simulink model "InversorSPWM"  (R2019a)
settings: Solver=ode23t  StartTime=0.0  StopTime=0.06  RelTol=1e-3
libraries: powerlib x22, powerlib_meascontrol x5, simulink x4

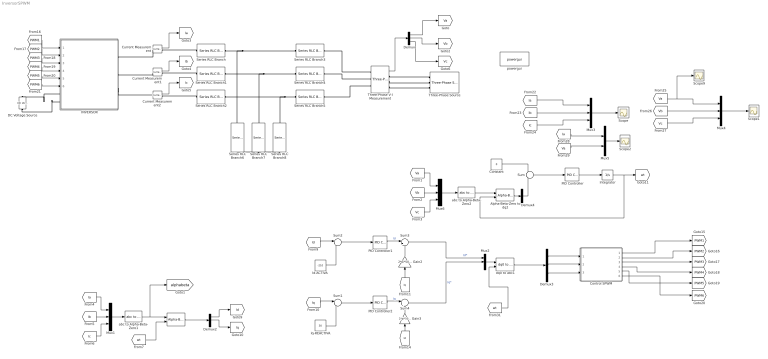
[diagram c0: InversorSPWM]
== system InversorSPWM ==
  " " : powerlib_meascontrol/Transformations/Alpha-Beta-Zero to dq0  Alignment=90 degrees behind phase A axis
  Alpha-Beta-Zero to dq2 : powerlib_meascontrol/Transformations/Alpha-Beta-Zero to dq0  Alignment=90 degrees behind phase A axis
  Constant : Constant  Value=0
  "Control SPWM " : Subsystem
  Current Measurement : powerlib/Measurements/Current Measurement  PhasorSimulation=off  OutputType=Complex  PSBequivalent=0
  Current Measurement1 : powerlib/Measurements/Current Measurement  PhasorSimulation=off  OutputType=Complex  PSBequivalent=0
  Current Measurement2 : powerlib/Measurements/Current Measurement  PhasorSimulation=off  OutputType=Complex  PSBequivalent=0
  DC Voltage Source : powerlib/Electrical Sources/DC Voltage Source  Amplitude=800  Measurements=None
  Demux{,2..4} (4 alike) : Demux  Outputs=3
  Gain2 : Gain  Gain=2*pi*50*1000e-6
  Gain3 : Gain  Gain=2*pi*50*1000e-6
  INVERSOR : Subsystem
  "Id-ACTIVA " : Constant  Value=-210
  Integrator : Integrator
  Iq-REACTIVA : Constant  Value=30
  Mux{1..4,6} (5 alike) : Mux  Inputs=3
  Mux5 : Mux  Inputs=2
  PID Controller : simulink/Continuous/PID Controller  Controller=PI  Form=Parallel  TimeDomain=Continuous-time  SampleTime=-1  IntegratorMethod=Forward Euler  FilterMethod=Forward Euler  ControllerParametersSource=internal  P=10  I=50000  D=0  UseFilter=on  N=100  TunerSelectOption=Transfer Function Based (PID Tuner App)  InitialConditionSource=internal  InitialConditionForIntegrator=0  InitialConditionForFilter=0  DifferentiatorICPrevScaledInput=0  ExternalReset=none  TrackingMode=off  Kt=1  LimitOutput=off  UpperSaturationLimit=inf  LowerSaturationLimit=-inf  LinearizeAsGain=on  AntiWindupMode=none  Kb=1  POutMin=[]  POutMax=[]  IOutMin=[]  IOutMax=[]  DOutMin=[]  DOutMax=[]  NOutMin=[]  NOutMax=[]  SumOutMin=[]  SumOutMax=[]  SaturationOutMin=[]  SaturationOutMax=[]  PParamMin=[]  PParamMax=[]  IParamMin=[]  IParamMax=[]  DParamMin=[]  DParamMax=[]  NParamMin=[]  NParamMax=[]  KbParamMin=[]  KbParamMax=[]  KtParamMin=[]  KtParamMax=[]  KbOutMin=[]  KbOutMax=[]  KtOutMin=[]  KtOutMax=[]  IntegratorOutMin=[]  IntegratorOutMax=[]  FilterOutMin=[]  FilterOutMax=[]  SumI1OutMin=[]  SumI1OutMax=[]  SumI2OutMin=[]  SumI2OutMax=[]  SumI3OutMin=[]  SumI3OutMax=[]  SumI4OutMin=[]  SumI4OutMax=[]  SumDOutMin=[]  SumDOutMax=[]  DifferentiatorOutMin=[]  DifferentiatorOutMax=[]  FilterDiffOutCoefMin=[]  FilterDiffOutCoefMax=[]  ReciprocalOutMin=[]  ReciprocalOutMax=[]  SumDenOutMin=[]  SumDenOutMax=[]  SumNumOutMin=[]  SumNumOutMax=[]  DivideOutMin=[]  DivideOutMax=[]  IntegratorContinuousStateAttributes=''  IntegratorStateMustResolveToSignalObject=off  IntegratorRTWStateStorageClass=Auto  FilterContinuousStateAttributes=''  FilterStateMustResolveToSignalObject=off  FilterRTWStateStorageClass=Auto  ParallelPVariant=InternalParameters  IdealPVariant=Disabled  IVariant=InternalParameters  DVariant=Disabled  IntegratorVariant=Continuous  SatVariant=Disabled  AWVariant=Passthrough  PCopyVariant=Disabled  TRVariant=Disabled  FdbkBlocksVariant=Forward  IdealPFdbkVariant=Disabled  SatFdbkVariant=Disabled  DerivativeFilterVariant=Disabled  NVariant=Disabled  NCopyVariant=Disabled_SignalSpec  FilterICVariant=Disabled  IntegratorICVariant=InternalICs  ExternalResetVariant=Disabled  TRSumVariant=Passthrough  SumFdbkVariant=Disabled  SumVariant=Sum_PI
  PID Controller1 : simulink/Continuous/PID Controller  Controller=PI  Form=Parallel  TimeDomain=Continuous-time  SampleTime=-1  IntegratorMethod=Forward Euler  FilterMethod=Forward Euler  ControllerParametersSource=internal  P=5  I=5000  D=0  UseFilter=on  N=100  TunerSelectOption=Transfer Function Based (PID Tuner App)  InitialConditionSource=internal  InitialConditionForIntegrator=0  InitialConditionForFilter=0  DifferentiatorICPrevScaledInput=0  ExternalReset=none  TrackingMode=off  Kt=1  LimitOutput=off  UpperSaturationLimit=inf  LowerSaturationLimit=-inf  LinearizeAsGain=on  AntiWindupMode=none  Kb=1  POutMin=[]  POutMax=[]  IOutMin=[]  IOutMax=[]  DOutMin=[]  DOutMax=[]  NOutMin=[]  NOutMax=[]  SumOutMin=[]  SumOutMax=[]  SaturationOutMin=[]  SaturationOutMax=[]  PParamMin=[]  PParamMax=[]  IParamMin=[]  IParamMax=[]  DParamMin=[]  DParamMax=[]  NParamMin=[]  NParamMax=[]  KbParamMin=[]  KbParamMax=[]  KtParamMin=[]  KtParamMax=[]  KbOutMin=[]  KbOutMax=[]  KtOutMin=[]  KtOutMax=[]  IntegratorOutMin=[]  IntegratorOutMax=[]  FilterOutMin=[]  FilterOutMax=[]  SumI1OutMin=[]  SumI1OutMax=[]  SumI2OutMin=[]  SumI2OutMax=[]  SumI3OutMin=[]  SumI3OutMax=[]  SumI4OutMin=[]  SumI4OutMax=[]  SumDOutMin=[]  SumDOutMax=[]  DifferentiatorOutMin=[]  DifferentiatorOutMax=[]  FilterDiffOutCoefMin=[]  FilterDiffOutCoefMax=[]  ReciprocalOutMin=[]  ReciprocalOutMax=[]  SumDenOutMin=[]  SumDenOutMax=[]  SumNumOutMin=[]  SumNumOutMax=[]  DivideOutMin=[]  DivideOutMax=[]  IntegratorContinuousStateAttributes=''  IntegratorStateMustResolveToSignalObject=off  IntegratorRTWStateStorageClass=Auto  FilterContinuousStateAttributes=''  FilterStateMustResolveToSignalObject=off  FilterRTWStateStorageClass=Auto  ParallelPVariant=InternalParameters  IdealPVariant=Disabled  IVariant=InternalParameters  DVariant=Disabled  IntegratorVariant=Continuous  SatVariant=Disabled  AWVariant=Passthrough  PCopyVariant=Disabled  TRVariant=Disabled  FdbkBlocksVariant=Forward  IdealPFdbkVariant=Disabled  SatFdbkVariant=Disabled  DerivativeFilterVariant=Disabled  NVariant=Disabled  NCopyVariant=Disabled_SignalSpec  FilterICVariant=Disabled  IntegratorICVariant=InternalICs  ExternalResetVariant=Disabled  TRSumVariant=Passthrough  SumFdbkVariant=Disabled  SumVariant=Sum_PI
  PID Controller2 : simulink/Continuous/PID Controller  Controller=PI  Form=Parallel  TimeDomain=Continuous-time  SampleTime=-1  IntegratorMethod=Forward Euler  FilterMethod=Forward Euler  ControllerParametersSource=internal  P=5  I=5000  D=0  UseFilter=on  N=100  TunerSelectOption=Transfer Function Based (PID Tuner App)  InitialConditionSource=internal  InitialConditionForIntegrator=0  InitialConditionForFilter=0  DifferentiatorICPrevScaledInput=0  ExternalReset=none  TrackingMode=off  Kt=1  LimitOutput=off  UpperSaturationLimit=inf  LowerSaturationLimit=-inf  LinearizeAsGain=on  AntiWindupMode=none  Kb=1  POutMin=[]  POutMax=[]  IOutMin=[]  IOutMax=[]  DOutMin=[]  DOutMax=[]  NOutMin=[]  NOutMax=[]  SumOutMin=[]  SumOutMax=[]  SaturationOutMin=[]  SaturationOutMax=[]  PParamMin=[]  PParamMax=[]  IParamMin=[]  IParamMax=[]  DParamMin=[]  DParamMax=[]  NParamMin=[]  NParamMax=[]  KbParamMin=[]  KbParamMax=[]  KtParamMin=[]  KtParamMax=[]  KbOutMin=[]  KbOutMax=[]  KtOutMin=[]  KtOutMax=[]  IntegratorOutMin=[]  IntegratorOutMax=[]  FilterOutMin=[]  FilterOutMax=[]  SumI1OutMin=[]  SumI1OutMax=[]  SumI2OutMin=[]  SumI2OutMax=[]  SumI3OutMin=[]  SumI3OutMax=[]  SumI4OutMin=[]  SumI4OutMax=[]  SumDOutMin=[]  SumDOutMax=[]  DifferentiatorOutMin=[]  DifferentiatorOutMax=[]  FilterDiffOutCoefMin=[]  FilterDiffOutCoefMax=[]  ReciprocalOutMin=[]  ReciprocalOutMax=[]  SumDenOutMin=[]  SumDenOutMax=[]  SumNumOutMin=[]  SumNumOutMax=[]  DivideOutMin=[]  DivideOutMax=[]  IntegratorContinuousStateAttributes=''  IntegratorStateMustResolveToSignalObject=off  IntegratorRTWStateStorageClass=Auto  FilterContinuousStateAttributes=''  FilterStateMustResolveToSignalObject=off  FilterRTWStateStorageClass=Auto  ParallelPVariant=InternalParameters  IdealPVariant=Disabled  IVariant=InternalParameters  DVariant=Disabled  IntegratorVariant=Continuous  SatVariant=Disabled  AWVariant=Passthrough  PCopyVariant=Disabled  TRVariant=Disabled  FdbkBlocksVariant=Forward  IdealPFdbkVariant=Disabled  SatFdbkVariant=Disabled  DerivativeFilterVariant=Disabled  NVariant=Disabled  NCopyVariant=Disabled_SignalSpec  FilterICVariant=Disabled  IntegratorICVariant=InternalICs  ExternalResetVariant=Disabled  TRSumVariant=Passthrough  SumFdbkVariant=Disabled  SumVariant=Sum_PI
  Scope{,1..2,9} (4 alike) : Scope
  Series RLC Branch{,1..5} (6 alike) : powerlib/Elements/Series RLC Branch  LConnTagsString=__new0  RConnTagsString=__new0  BranchType=L  Resistance=1  Inductance=500e-6  SetiL0=off  InitialCurrent=0  Capacitance=1e-6  Setx0=off  InitialVoltage=0  Measurements=None
  Series RLC Branch6 : powerlib/Elements/Series RLC Branch  LConnTagsString=__new0  RConnTagsString=__new0  BranchType=C  Resistance=1  Inductance=500e-6  SetiL0=off  InitialCurrent=0  Capacitance=100e-9  Setx0=off  InitialVoltage=0  Measurements=None
  Series RLC Branch7 : powerlib/Elements/Series RLC Branch  LConnTagsString=__new0  RConnTagsString=__new0  BranchType=C  Resistance=1  Inductance=500e-6  SetiL0=off  InitialCurrent=0  Capacitance=100e-9  Setx0=off  InitialVoltage=0  Measurements=None
  Series RLC Branch8 : powerlib/Elements/Series RLC Branch  LConnTagsString=__new0  RConnTagsString=__new0  BranchType=C  Resistance=1  Inductance=500e-6  SetiL0=off  InitialCurrent=0  Capacitance=100e-9  Setx0=off  InitialVoltage=0  Measurements=None
  Sum : Sum  Inputs=+-
  Sum1 : Sum  Inputs=|-+
  Sum2 : Sum  Inputs=|-+
  Sum3 : Sum  Inputs=|++
  Sum4 : Sum  Inputs=|+-
  Three-Phase V-I Measurement : powerlib/Measurements/Three-Phase V-I Measurement  VoltageMeasurement=phase-to-phase  SetLabelV=off  LabelV=Vabc  Vpu=off  VpuLL=off  CurrentMeasurement=no  SetLabelI=off  LabelI=Iabc  Ipu=off  Pbase=100e6  Vbase=500e3  OutputType=Complex  PhasorSimulation=off  PSBequivalent=0
  Three-Phase Source : powerlib/Electrical Sources/Three-Phase Source  InternalConnection=Y  VoltagePhases=off  Voltage=415  PhaseAngle=0  Voltage_phases=[25e3 25e3 25e3]/sqrt(3)  PhaseAngles_phases=[0 -120 +120]  Frequency=50  NonIdealSource=on  SpecifyImpedance=off  Resistance=0.001e-3  Inductance=0.001e-9  ShortCircuitLevel=100e6  BaseVoltage=415  XRratio=7  BusType=swing  Pref=10e3  Qref=0  Prefabc=[10e3, 10e3, 10e3]  Qrefabc=[0, 0, 0]  Qmin=-inf  Qmax=inf
  abc to Alpha-Beta-Zero1 : powerlib_meascontrol/Transformations/abc to Alpha-Beta-Zero
  abc to Alpha-Beta-Zero2 : powerlib_meascontrol/Transformations/abc to Alpha-Beta-Zero
  dq0 to abc1 : powerlib_meascontrol/Transformations/dq0 to abc  Alignment=90 degrees behind phase A axis
  powergui : powerlib/powergui  Priority=1  SimulationMode=Discrete  SampleTime=1e-6  frequency=60  Iterations=50  frequencyindice=50  Pbase=100e6  ErrMax=1e-4  UnitsV=kV  UnitsW=MW  buscounter=0  FunctionMessages=off  echomessages=off  EnableUseOfTLC=off  CurrentSourceSwitches=off  DisableSnubberDevices=off  DisableRonSwitches=off  DisableVfSwitches=off  DisplayEquations=off  AutomaticDiscreteSolvers=off  SolverType=Tustin/Backward Euler (TBE)  Interpol=off  ExternalGateDelay=off  methode=off  Ts=100  x0status=blocks  SPID=on  SwTol=0  HookPort=off  NonlinearTolerance=0  nMaxIteration=15  ContinueOnMaxIteration=off  RestoreLinks=warning  ResistiveCurrentMeasurement=off  Frange=[0:2:500]  Ylog=off  Xlog=on  ShowGrid=off  save=off  variable=ZData  structure=0  ZoomFFT=off  StartTime=0.0  cycles=1  DisplayStyle=1  fundamental=60  FreqAxis=off  MaxFrequency=1000  frequencyindicesteady=1  RmsSteady=1  display=off
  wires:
  [PWM6] -> INVERSOR/6(PWM6)
  [PWM2] -> INVERSOR/2(PWM2)
  [PWM5] -> INVERSOR/5(PWM5)
  [PWM3] -> INVERSOR/3(PWM3)
  Sum4/1 -> Mux2/2  "Iq*"
  Sum3/1 -> Mux2/1  "Id*"
  [Id] -> Gain3/1
  Current Measurement/1 -> [Ia]
  Sum1/1 -> PID Controller2/1
  PID Controller2/1 -> Sum4/1  "Iq"
  Iq-REACTIVA/1 -> Sum1/2
  [Id] -> Sum2/1
  Integrator/1 -> Alpha-Beta-Zero to dq2/2, [wt]
  PID Controller/1 -> Integrator/1
  " "/1 -> Demux2/1
  [Ib] -> Mux1/2
  Demux2/1 -> [Id]
  [Ic] -> Mux1/3
  Mux1/1 -> abc to Alpha-Beta-Zero1/1
  Sum2/1 -> PID Controller1/1
  [Ia] -> Mux1/1
  Demux2/2 -> [Iq]
  [wt] -> " "/2
  [Iq] -> Gain2/1
  Current Measurement2/1 -> [Ic]
  Current Measurement1/1 -> [Ib]
  Gain3/1 -> Sum4/2
  PID Controller1/1 -> Sum3/1  "Id"
  abc to Alpha-Beta-Zero2/1 -> Alpha-Beta-Zero to dq2/1
  Constant/1 -> Sum/1
  Sum/1 -> PID Controller/1
  [PWM4] -> INVERSOR/4(PWM4)
  [PWM1] -> INVERSOR/1(PWM1)
  Gain2/1 -> Sum3/2
  "Id-ACTIVA "/1 -> Sum2/2
  [Iq] -> Sum1/1
  Demux3/1 -> "Control SPWM "/1("Ia ")
  Demux3/2 -> "Control SPWM "/2("Ib ")
  Demux3/3 -> "Control SPWM "/3(Ic)
  "Control SPWM "/5(PWM5) -> [PWM5]
  "Control SPWM "/1("PWM1 ") -> [PWM1]
  "Control SPWM "/4(PWM4) -> [PWM4]
  "Control SPWM "/6(PWM6) -> [PWM6]
  "Control SPWM "/3(PWM3) -> [PWM3]
  "Control SPWM "/2("PWM2 ") -> [PWM2]
  [Ic] -> Mux3/3
  [Ib] -> Mux3/2
  Mux3/1 -> Scope/1
  Mux4/1 -> Scope1/1
  [Va] -> Scope9/1, Mux4/1
  [Vb] -> Mux4/2
  [Vc] -> Mux4/3
  Alpha-Beta-Zero to dq2/1 -> Demux4/1
  Demux4/2 -> Sum/2
  [Ia] -> Mux5/1
  [Va] -> Mux5/2
  Mux5/1 -> Scope2/1
  dq0 to abc1/1 -> Demux3/1
  Mux2/1 -> dq0 to abc1/1
  [wt] -> dq0 to abc1/2
  [Ia] -> Mux3/1
  abc to Alpha-Beta-Zero1/1 -> [alphabeta], " "/1
  Three-Phase V-I Measurement/1 -> Demux/1
  Demux/3 -> [Vc]
  Demux/2 -> [Vb]
  Demux/1 -> [Va]
  [Va] -> Mux6/1
  [Vb] -> Mux6/2
  [Vc] -> Mux6/3
  Mux6/1 -> abc to Alpha-Beta-Zero2/1
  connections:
  Series RLC Branch7/RConn1 -- Series RLC Branch6/RConn1 -- Series RLC Branch8/RConn1
  Series RLC Branch5/LConn1 -- Series RLC Branch8/LConn1 -- Series RLC Branch2/RConn1
  Series RLC Branch4/LConn1 -- Series RLC Branch7/LConn1 -- Series RLC Branch1/RConn1
  Series RLC Branch3/LConn1 -- Series RLC Branch6/LConn1 -- Series RLC Branch/RConn1
  Three-Phase V-I Measurement/RConn3 -- Three-Phase Source/RConn3
  Series RLC Branch/LConn1 -- Current Measurement/RConn1
  Series RLC Branch2/LConn1 -- Current Measurement2/RConn1
  Series RLC Branch1/LConn1 -- Current Measurement1/RConn1
  Current Measurement/LConn1 -- INVERSOR/RConn1
  Current Measurement1/LConn1 -- INVERSOR/RConn2
  DC Voltage Source/LConn1 -- INVERSOR/LConn2
  DC Voltage Source/RConn1 -- INVERSOR/LConn1
  INVERSOR/RConn3 -- Current Measurement2/LConn1
  Series RLC Branch3/RConn1 -- Three-Phase V-I Measurement/LConn1
  Series RLC Branch4/RConn1 -- Three-Phase V-I Measurement/LConn2
  Three-Phase V-I Measurement/RConn1 -- Three-Phase Source/RConn1
  Three-Phase V-I Measurement/RConn2 -- Three-Phase Source/RConn2
  Series RLC Branch5/RConn1 -- Three-Phase V-I Measurement/LConn3

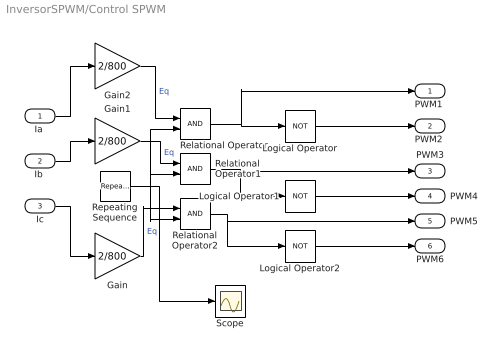
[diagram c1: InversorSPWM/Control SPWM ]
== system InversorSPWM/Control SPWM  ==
  "Ia " : Inport
  "Ib " : Inport  Port=2
  Ic : Inport  Port=3
  Gain : Gain  Gain=2/800
  Gain1 : Gain  Gain=2/800
  Gain2 : Gain  Gain=2/800
  Logical Operator : Logic  Operator=NOT  AllPortsSameDT=off  OutDataTypeStr=boolean
  Logical Operator1 : Logic  Operator=NOT  AllPortsSameDT=off  OutDataTypeStr=boolean
  Logical Operator2 : Logic  Operator=NOT  AllPortsSameDT=off  OutDataTypeStr=boolean
  Relational Operator : RelationalOperator  OutDataTypeStr=boolean  RndMeth=Simplest
  Relational Operator1 : RelationalOperator  OutDataTypeStr=boolean  RndMeth=Simplest
  Relational Operator2 : RelationalOperator  OutDataTypeStr=boolean  RndMeth=Simplest
  Repeating Sequence : simulink/Sources/Repeating Sequence  rep_seq_t=[0 0.00005 0.0001]  rep_seq_y=[-1 1 -1]
  Scope : Scope
  "PWM1 " : Outport
  "PWM2 " : Outport  Port=2
  PWM3 : Outport  Port=3
  PWM4 : Outport  Port=4
  PWM5 : Outport  Port=5
  PWM6 : Outport  Port=6
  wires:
  Relational Operator/1 -> "PWM1 "/1, Logical Operator/1
  Relational Operator2/1 -> Logical Operator2/1, PWM5/1
  "Ia "/1 -> Gain2/1
  Relational Operator1/1 -> Logical Operator1/1, PWM3/1
  Ic/1 -> Gain/1
  Repeating Sequence/1 -> Scope/1, Relational Operator2/2, Relational Operator1/2, Relational Operator/2
  "Ib "/1 -> Gain1/1
  Logical Operator/1 -> "PWM2 "/1
  Logical Operator1/1 -> PWM4/1
  Logical Operator2/1 -> PWM6/1
  Gain/1 -> Relational Operator2/1  "Eq"
  Gain1/1 -> Relational Operator1/1  "Eq"
  Gain2/1 -> Relational Operator/1  "Eq"

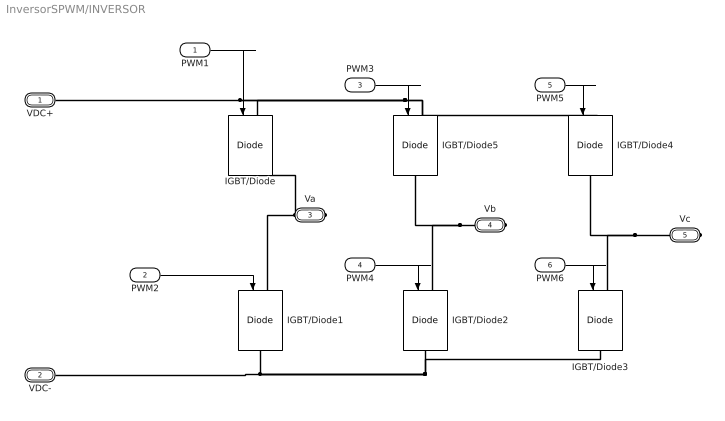
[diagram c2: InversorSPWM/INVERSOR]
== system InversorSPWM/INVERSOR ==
  PWM1 : Inport
  PWM2 : Inport  Port=2
  PWM3 : Inport  Port=3
  PWM4 : Inport  Port=4
  PWM5 : Inport  Port=5
  PWM6 : Inport  Port=6
  IGBT/Diode{,1..5} (6 alike) : powerlib/Power Electronics/IGBT//Diode  Ron=1e-3  Rs=1e5  Cs=inf  Measurements=off
  VDC+ : PMIOPort  Side=Left
  VDC- : PMIOPort  Port=2  Side=Left
  Va : PMIOPort  Port=3  Side=Right
  Vb : PMIOPort  Port=4  Side=Right
  Vc : PMIOPort  Port=5  Side=Right
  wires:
  PWM6/1 -> IGBT/Diode3/1
  PWM4/1 -> IGBT/Diode2/1
  PWM5/1 -> IGBT/Diode4/1
  PWM1/1 -> IGBT/Diode/1
  PWM2/1 -> IGBT/Diode1/1
  PWM3/1 -> IGBT/Diode5/1
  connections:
  IGBT/Diode/LConn1 -- VDC+/RConn1 -- IGBT/Diode5/LConn1 -- IGBT/Diode4/LConn1
  IGBT/Diode1/RConn1 -- VDC-/RConn1 -- IGBT/Diode3/RConn1 -- IGBT/Diode2/RConn1
  Vb/RConn1 -- IGBT/Diode5/RConn1 -- IGBT/Diode2/LConn1
  Vc/RConn1 -- IGBT/Diode4/RConn1 -- IGBT/Diode3/LConn1
  Va/RConn1 -- IGBT/Diode1/LConn1 -- IGBT/Diode/RConn1
